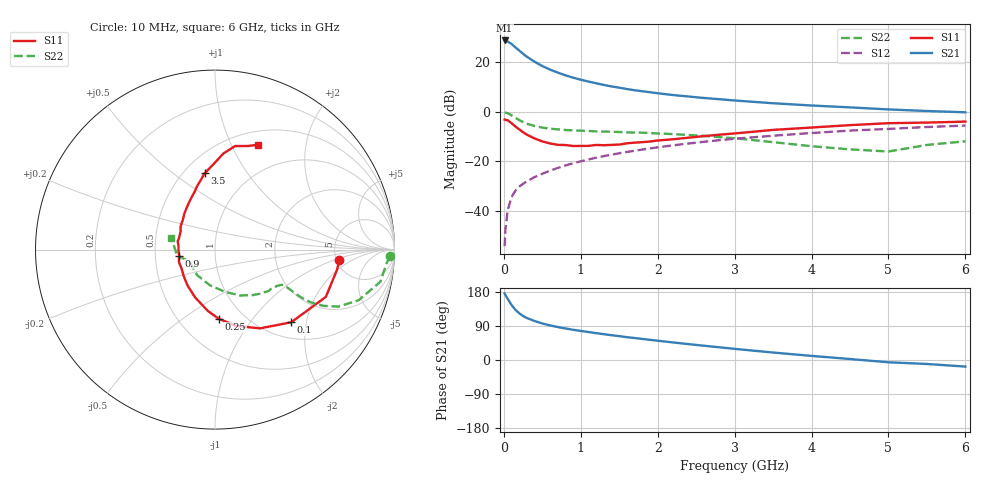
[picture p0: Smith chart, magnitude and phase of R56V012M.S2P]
! SIEMENS Small Signal Semiconductors
! BFR183
! Si NPN RF Bipolar Junction Transistor in SOT23
! VCE = 6 V  IC = 12 mA
! Common Emitter S-Parameters:  May  1996
# GHz  S  MA  R  50
!  f  S11  S21  S12  S22
! GHz  MAG  ANG  MAG  ANG  MAG  ANG  MAG  ANG
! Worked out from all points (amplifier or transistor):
!   36 points, 10 MHz to 6 GHz, reference 50 ohm
!   highest |S21| = 28.9 dB at 10 MHz (marker M1)
!   |S21| within 3 dB of that: start of sweep to 158.1 MHz
!   unconditionally stable (mu >= 1): 754 MHz to 2.544 GHz
!   at 250 MHz: K = 0.66, MSG = 26.3 dB, |S12| = -29.2 dB
!   at 1.4 GHz: K = 1.05, MAG = 12.4 dB, |S12| = -17.4 dB
!   at 6 GHz: K = 0.89, MSG = 2.7 dB, |S12| = -5.6 dB
!   S11 on the Smith chart (normalised r, x): 10 MHz: 5.29, -1.19; 100 MHz: 1.33, -1.64; 250 MHz: 0.77, -0.70; 900 MHz: 0.67, -0.05; 3.5 GHz: 0.63, +0.66; 6 GHz: 0.65, +1.28
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0.01  0.6956 -4.8  27.85 175.8  0.0019 92.7  0.9749 -2.2
0.02  0.6889 -9.5  27.49 171.8  0.004 86.6  0.9597 -4.5
0.05  0.6713 -23.1  26.55 161.2  0.0103 78.7  0.9386 -11.0
0.1  0.5869 -43.6  23.69 145.3  0.0186 72.2  0.8488 -19.4
0.15  0.5053 -60.3  20.21 132.5  0.0253 67.5  0.7569 -24.8
0.2  0.4414 -74.4  17.37 123.4  0.0305 64.8  0.6809 -27.4
0.25  0.3862 -86.8  14.94 116.1  0.0348 64.7  0.6186 -28.7
0.3  0.3441 -96.7  13.04 110.7  0.0393 65.1  0.5733 -29.1
0.4  0.2884 -112.6  10.31 102.9  0.0476 65.1  0.5158 -28.8
0.5  0.2513 -127.7  8.443 96.3  0.0556 66.1  0.4786 -28.1
0.6  0.2288 -139.5  7.174 91.4  0.0643 66.3  0.4556 -27.7
0.7  0.2142 -150.5  6.234 87.0  0.0728 67.3  0.4406 -27.5
0.9  0.2028 -170.4  4.91 79.8  0.0908 67.0  0.4203 -27.8
1.1  0.2042 174.2  4.097 73.8  0.1083 66.5  0.4082 -29.4
1.3  0.2104 162.3  3.499 68.1  0.1266 65.7  0.3975 -30.9
1.6  0.2302 146.1  2.885 60.2  0.1538 63.5  0.383 -34.7
2.2  0.278 125.2  2.183 46.3  0.2093 58.4  0.3541 -43.9
3.5  0.4302 97.5  1.49 19.7  0.3279 43.3  0.2427 -76.3
4.5  0.537 85.1  1.228 2.6  0.4167 31.1  0.1735 -125.2
5  0.5877 79.0  1.117 -6.0  0.4504 23.8  0.157 -155.1
5.5  0.605 72.5  1.038 -10.5  0.4918 19.6  0.2131 -171.2
6  0.6327 67.5  0.977 -17.4  0.527 12.0  0.2527 164.7
